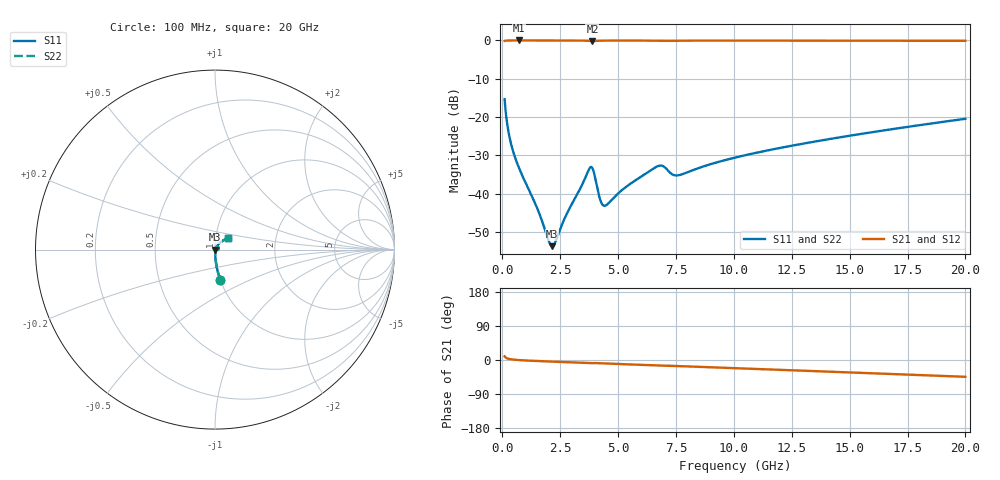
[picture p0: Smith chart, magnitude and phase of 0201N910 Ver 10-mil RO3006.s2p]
# GHz S MA R 50
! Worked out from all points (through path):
!   1601 points, 100 MHz to 20 GHz, reference 50 ohm
!   highest |S21| = -0.01 dB at 709.4 MHz (marker M1); lowest = -0.2 dB at 3.893 GHz (marker M2)
!   group delay of S21, straight-line fit = 6.27 ps
!   lowest |S11| = -53.7 dB at 2.152 GHz (marker M3), VSWR 1.00, Z = 50.2 - j0.0357 ohm
!   |S11| at or under -10 dB: start of sweep to end of sweep
!   |S22| runs from -53.7 to -15.3 dB; largest |S21 - S12| = 0
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0.1  0.1715 -80.1  0.9845 9.7  0.9845 9.7  0.1715 -80.1
0.2616875  0.06563 -86.1  0.9971 3.2  0.9971 3.2  0.06563 -86.1
0.3611875  0.04702 -87.0  0.9981 2.0  0.9981 2.0  0.04702 -87.0
0.7094375  0.02216 -87.4  0.9987 -0.2  0.9987 -0.2  0.02216 -87.4
1.517875  0.006356 -77.6  0.9983 -2.7  0.9983 -2.7  0.006356 -77.6
2.015375  0.002383 -38.0  0.998 -4.0  0.998 -4.0  0.002383 -38.0
2.152188  0.002074 -9.9  0.9979 -4.3  0.9979 -4.3  0.002074 -9.9
2.289  0.002336 17.8  0.9978 -4.6  0.9978 -4.6  0.002336 17.8
2.749188  0.005204 54.7  0.9974 -5.8  0.9974 -5.8  0.005204 54.7
3.420812  0.01262 59.8  0.995 -7.5  0.995 -7.5  0.01262 59.8
3.756625  0.0212 38.1  0.9852 -8.4  0.9852 -8.4  0.0212 38.1
3.893438  0.02157 12.9  0.9797 -8.2  0.9797 -8.2  0.02157 12.9
4.22925  0.008343 0.7  0.9917 -8.5  0.9917 -8.5  0.008343 0.7
4.42825  0.006983 25.3  0.9941 -9.1  0.9941 -9.1  0.006983 25.3
5.398375  0.01265 59.4  0.9956 -11.5  0.9956 -11.5  0.01265 59.4
6.741625  0.02305 49.6  0.9896 -14.6  0.9896 -14.6  0.02305 49.6
6.940625  0.02295 41.5  0.987 -14.9  0.987 -14.9  0.02295 41.5
7.574937  0.01738 46.7  0.9917 -16.0  0.9917 -16.0  0.01738 46.7
10.05  0.02962 58.7  0.9943 -21.6  0.9943 -21.6  0.02962 58.7
13.37081  0.04724 54.2  0.993 -29.1  0.993 -29.1  0.04724 54.2
16.69162  0.06859 48.2  0.991 -36.6  0.991 -36.6  0.06859 48.2
20  0.09499 41.5  0.9881 -44.3  0.9881 -44.3  0.09499 41.5
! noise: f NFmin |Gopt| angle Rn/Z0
0.1  0.0005161  0.9174  0.2374  0.00138
2.301  0.004421  0.7928  4.605  0.004396
4.515  0.009619  0.8116  9.019  0.01058
6.729  0.01608  0.8308  13.4  0.01976
8.943  0.01334  0.7433  17.72  0.01019
11.14  0.01494  0.72  21.98  0.01019
13.36  0.01696  0.7085  26.2  0.01088
15.57  0.01902  0.7008  30.37  0.01162
17.79  0.02106  0.6953  34.46  0.01234
20  0.0231  0.6915  38.49  0.01305
